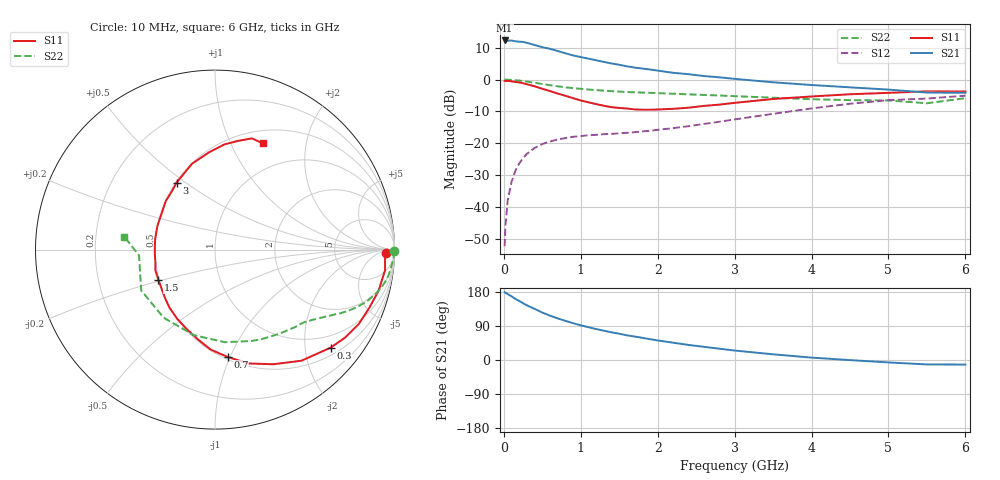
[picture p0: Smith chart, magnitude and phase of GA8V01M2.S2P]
! Infineon Technologies  Discrete & RF Semiconductors
! BF775
! Si NPN RF Bipolar Junction Transistor in SOT23
! VCE = 8 V  IC = 1.2 mA
! Common Emitter S-Parameters:  May  1996
# GHz  S  MA  R  50
!  f  S11  S21  S12  S22
! GHz  MAG  ANG  MAG  ANG  MAG  ANG  MAG  ANG
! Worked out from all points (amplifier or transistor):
!   36 points, 10 MHz to 6 GHz, reference 50 ohm
!   highest |S21| = 12.3 dB at 10 MHz (marker M1)
!   |S21| within 3 dB of that: start of sweep to 653.8 MHz
!   unconditionally stable (mu >= 1): 1.395 GHz to 3.425 GHz; 5.458 GHz to 5.595 GHz
!   at 250 MHz: K = 0.21, MSG = 18.3 dB, |S12| = -24.7 dB
!   at 1.4 GHz: K = 1.00, MAG = 10.7 dB, |S12| = -17.1 dB
!   at 6 GHz: K = 0.98, MSG = 0.5 dB, |S12| = -5.1 dB
!   S11 on the Smith chart (normalised r, x): 10 MHz: 35, -17; 300 MHz: 0.67, -2.57; 700 MHz: 0.52, -0.98; 1.5 GHz: 0.50, -0.19; 3 GHz: 0.50, +0.46; 6 GHz: 0.65, +1.33
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0.01  0.9551 -1.3  4.125 179.1  0.0024 89.2  0.9999 -0.5
0.02  0.9489 -2.9  4.123 177.4  0.0049 86.2  0.9967 -1.1
0.05  0.9545 -6.9  4.089 174.0  0.0126 84.3  0.9961 -2.8
0.1  0.9397 -14.1  4.111 168.1  0.0246 82.5  0.9867 -5.4
0.15  0.9187 -20.7  4.008 161.3  0.0368 77.4  0.9785 -8.3
0.25  0.875 -34.1  3.915 149.8  0.0582 69.6  0.9488 -13.1
0.3  0.8447 -40.3  3.789 144.2  0.0679 66.4  0.9293 -15.3
0.5  0.7164 -63.1  3.237 125.2  0.0968 55.2  0.8531 -22.1
0.6  0.6612 -73.6  3.043 117.1  0.1065 50.7  0.8159 -24.7
0.7  0.6026 -83.2  2.819 109.8  0.1141 47.7  0.7842 -26.9
0.9  0.5103 -100.6  2.4 97.2  0.126 42.9  0.7347 -30.2
1.1  0.4388 -118.9  2.137 86.6  0.133 40.6  0.6981 -33.1
1.3  0.3878 -135.9  1.897 77.4  0.1385 39.9  0.6694 -35.7
1.5  0.3581 -151.7  1.711 69.4  0.1428 40.6  0.6474 -38.4
1.9  0.3358 176.6  1.441 54.9  0.1567 43.3  0.6192 -44.5
2.2  0.3468 157.8  1.278 45.6  0.1723 46.0  0.5993 -49.6
3  0.4306 119.8  1.027 25.0  0.2362 49.3  0.5489 -68.0
3.5  0.4952 105.0  0.907 15.0  0.2894 47.4  0.519 -83.9
4.5  0.588 85.0  0.755 -0.3  0.417 36.6  0.4752 -126.9
5  0.6188 78.1  0.696 -6.4  0.4746 28.5  0.4702 -151.0
5.5  0.653 71.6  0.625 -11.7  0.5029 19.0  0.4245 -175.6
6  0.6491 65.8  0.62 -12.0  0.5585 14.0  0.5101 171.9
